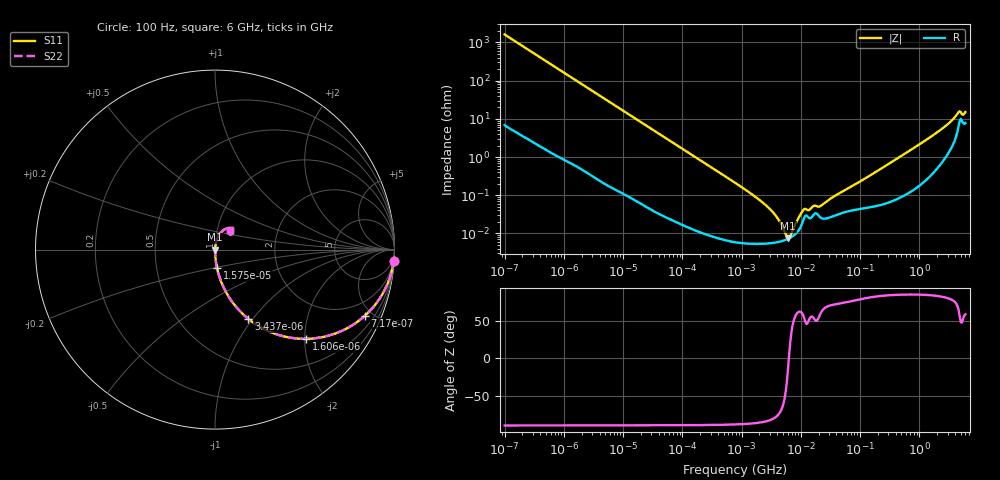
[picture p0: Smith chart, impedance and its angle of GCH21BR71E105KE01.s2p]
!Murata Part Number: GCH21BR71E105KE01
!These Parameters are Measured in Series Mode Connection
!Data Generated on Jun 19, 2026
!  o--ll--o
!Port1  Port2
!  o------o
!Operation Temp=25[degC], DC Bias Voltage=0[V]
!Freq. Start=100[Hz] Stop=6[GHz] 401[Steps]
# Hz S RI R 50
!Freq.(Hz) S11(Real) S11(Imag) S21(Real) S21(Imag) S12(Real) S12(Imag) S22(Real) S22(Imag)
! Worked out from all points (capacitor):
!   401 points, 100 Hz to 6 GHz, reference 50 ohm
!   read as one part in series: C = 984 nF near 109 Hz
!   lowest |Z| = 7.43 mohm at 6.075 MHz (marker M1)
!   series resonance near 6.282 MHz, so ESL is about 650 pH
!   S11 on the Smith chart (normalised r, x): 100 Hz: 1, -32; 717 Hz: 1.02, -4.53; 1.606 kHz: 1.01, -2.03; 3.437 kHz: 1.01, -0.95; 15.75 kHz: 1.00, -0.21; 6 GHz: 1.16, +0.26
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100  0.9959 -0.0617  0.00408 0.0617  0.00408 0.0617  0.9959 -0.0617
335  0.9582 -0.198  0.0418 0.198  0.0418 0.198  0.9582 -0.198
717  0.8355 -0.3683  0.1645 0.3683  0.1645 0.3683  0.8355 -0.3683
1606  0.5069 -0.4971  0.4931 0.4971  0.4931 0.4971  0.5069 -0.4971
2008  0.3975 -0.4865  0.6025 0.4865  0.6025 0.4865  0.3975 -0.4865
3437  0.1855 -0.3858  0.8145 0.3858  0.8145 0.3858  0.1855 -0.3858
6433  0.062 -0.2382  0.938 0.2382  0.938 0.2382  0.062 -0.2382
15752  0.0115 -0.103  0.9885 0.103  0.9885 0.103  0.0115 -0.103
40335  0.00199 -0.0408  0.998 0.0408  0.998 0.0408  0.00199 -0.0408
774597  6.34e-05 -0.00213  0.9999 0.00213  0.9999 0.00213  6.34e-05 -0.00213
2837864  5.5e-05 -0.000472  0.9999 0.000472  0.9999 0.000472  5.5e-05 -0.000472
4060267  5.93e-05 -0.000243  0.9999 0.000243  0.9999 0.000243  5.93e-05 -0.000243
5311619  6.63e-05 -9.18e-05  0.9999 9.18e-05  0.9999 9.18e-05  6.63e-05 -9.18e-05
6075234  7.2e-05 -1.83e-05  0.9999 1.83e-05  0.9999 1.83e-05  7.2e-05 -1.83e-05
7266822  8.42e-05 8.2e-05  0.9999 -8.2e-05  0.9999 -8.2e-05  8.42e-05 8.2e-05
1.087309e7  0.000209 0.00034  0.9998 -0.00034  0.9998 -0.00034  0.000209 0.00034
1.555665e7  0.000273 0.000405  0.9997 -0.000405  0.9997 -0.000405  0.000273 0.000405
2.225763e7  0.000252 0.000478  0.9997 -0.000478  0.9997 -0.000478  0.000252 0.000478
3.124326e8  0.000699 0.00675  0.9993 -0.00675  0.9993 -0.00675  0.000699 0.00675
2.048624e9  0.00719 0.0446  0.9928 -0.0446  0.9928 -0.0446  0.00719 0.0446
4.586474e9  0.0729 0.1179  0.9271 -0.1179  0.9271 -0.1179  0.0729 0.1179
6e9  0.0853 0.1097  0.9147 -0.1097  0.9147 -0.1097  0.0853 0.1097
